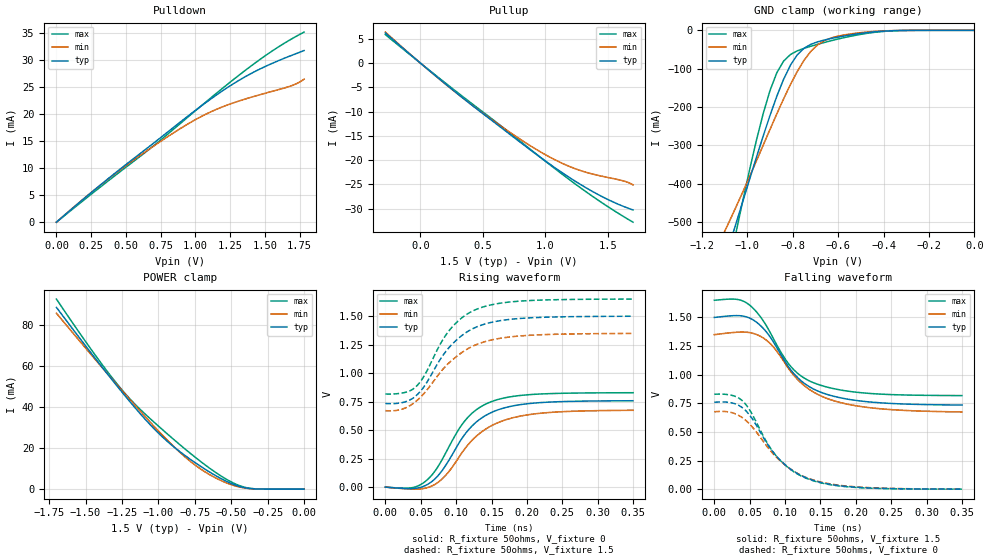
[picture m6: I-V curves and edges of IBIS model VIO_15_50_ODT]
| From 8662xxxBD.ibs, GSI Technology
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[Model]   VIO_15_50_ODT
Model_type   I/O
Polarity   Non-Inverting
Vinl  =   0.5500V
Vinh  =   0.9500V
Vmeas =   0.75v
Rref  =   50
|  variable   typ   min   max
C_comp   3.0pF   2.5pF   3.5pF
[Receiver Thresholds]
Vth = 0.75V
Vth_min = 0.68V
Vth_max = 0.825V
Threshold_sensitivity = 1.0
Reference_supply Ext_ref
Vinh_ac = +200mv
Vinh_dc = +100mv
Vinl_ac = -200mv
Vinl_dc = -100mv
Tslew_ac = 550ps
|  variable   typ   min   max
[External Reference]   0.75   0.68   0.825
|  variable   typ   min   max
[Temperature Range]   50   100   0
|  variable   typ   min   max
[Voltage Range]   1.5   1.35   1.65
[Add Submodel]
| Submodel Name   Mode
Strong_ODT_18V   Non-Driving
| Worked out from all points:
|   slope of the pulldown table from 0 to 0.225 V, typ, clamps not added: 45.5 ohm
|   slope of the pullup table from 0 to 0.225 V, typ, clamps not added: 46.7 ohm
|   GND clamp passes 1 mA (typ) near -0.36 V on its own axis
|   POWER clamp passes 1 mA (typ) near -0.42 V on its own axis
|   rising waveform, R_fixture 50ohms, V_fixture 0: 20-80 % time 55.1ps typ, 60.6ps min, 52.3ps max; typ from 0 V to 0.757 V
|   rising waveform, R_fixture 50ohms, V_fixture 1.5: 20-80 % time 56.4ps typ, 63.8ps min, 52.1ps max; typ from 0.733 V to 1.5 V
|   falling waveform, R_fixture 50ohms, V_fixture 1.5: 20-80 % time 59.4ps typ, 65.4ps min, 56ps max; typ from 1.5 V to 0.735 V
|   falling waveform, R_fixture 50ohms, V_fixture 0: 20-80 % time 58.8ps typ, 64.2ps min, 56.4ps max; typ from 0.759 V to 0 V
[Pullup]
| V(VDDQ-Vout)   typ   min   max
-280mV    6.194mA    6.382mA    5.865mA
40mV      -869.6uA   -882.7uA   -829.9uA
340mV     -7.204mA   -7.213mA   -6.928mA
620mV     -12.79mA   -12.56mA   -12.46mA
900mV     -18.3mA    -17.38mA   -18.2mA
1.08V     -21.65mA   -19.99mA   -21.84mA
1.24V     -24.38mA   -21.79mA   -24.95mA
1.34V     -25.93mA   -22.62mA   -26.8mA
1.48V     -27.87mA   -23.47mA   -29.27mA
1.62V     -29.5mA    -24.26mA   -31.56mA
1.7V      -30.27mA   -25.11mA   -32.79mA
[PullDown]
| voltage   typ   min   max
0V        -6.62nA    -14.14nA   -2.867nA
252mV     5.521mA    5.53mA     5.214mA
468mV     10.03mA    9.889mA    9.552mA
774mV     16.17mA    15.4mA     15.75mA
972mV     20.17mA    18.6mA     20.04mA
1.152V    23.59mA    20.93mA    23.91mA
1.368V    27.1mA     22.9mA     28.32mA
1.53V     29.18mA    24.1mA     31.34mA
1.674V    30.74mA    25.14mA    33.7mA
1.728V    31.28mA    25.68mA    34.49mA
1.782V    31.82mA    26.51mA    35.24mA
[POWER Clamp]
|V(VDDQ-Vout)   typ   min   max
-1.7V     88.47mA    85.63mA    92.51mA
-1.428V   63.15mA    62.67mA    64.71mA
-1.224V   45.01mA    45.89mA    46.19mA
-1.122V   36.5mA     37.74mA    38.64mA
-1.02V    28.71mA    29.85mA    31.98mA
-918mV    21.99mA    22.38mA    25.61mA
-816mV    16.3mA     15.63mA    19.48mA
-646mV    8.221mA    6.972mA    10.07mA
-544mV    4.192mA    3.378mA    5.259mA
-442mV    1.292mA    1.001mA    1.675mA
-340mV    147uA      124.8uA    177uA
0V        29.63nA    52.34nA    12.42nA
[GND Clamp]
|(Vout)   typ   min   max
-1.5V     -1.252A    -991.4mA   -1.695A
-1.11V    -618mA     -537.1mA   -698.9mA
-1.08V    -561.6mA   -499.5mA   -613mA
-1.05V    -504.3mA   -461mA     -527.9mA
-930mV    -275.4mA   -299.5mA   -216.7mA
-900mV    -221.7mA   -258.3mA   -156.7mA
-870mV    -171.8mA   -217.7mA   -110.4mA
-810mV    -90.75mA   -141.1mA   -63.05mA
-720mV    -36.4mA    -54.51mA   -41.47mA
-630mV    -21.2mA    -19.75mA   -26.98mA
-390mV    -1.825mA   -1.274mA   -2.426mA
0V        -6.62nA    -14.14nA   -2.873nA
[Ramp]
| voltage   typ   min   max
dV/dt_r   0.54/186p   0.48/213p   0.60/209p
dV/dt_f   0.86/129p   0.66/166p   1.07/101p
R_load  =   50ohms
[Rising Waveform]
R_fixture =   50ohms
V_fixture =   0
| Time   V(typ)   V(min)   V(max)
0s        156.2nV    330.9nV    69.99nV
38.5ps    -12.6mV    -17.51mV   -3.974mV
63ps      37.07mV    2.813mV    87.25mV
84ps      178.8mV    95.17mV    284.9mV
112ps     460.4mV    333.9mV    578.9mV
129.5ps   575.8mV    451.7mV    682.8mV
150.5ps   656.1mV    540.2mV    750.9mV
178.5ps   710mV      605.5mV    793.7mV
217ps     740.1mV    646.3mV    815.9mV
350ps     757.4mV    673.7mV    827.7mV
[Rising Waveform]
R_fixture =   50ohms
V_fixture =   1.5
V_fixture_min =  1.35
V_fixture_max =  1.65
| Time   V(typ)   V(min)   V(max)
0s        733.1mV    670.5mV    816.7mV
21ps      737.8mV    679mV      822.5mV
42ps      793.7mV    745.8mV    873.6mV
52.5ps    862.7mV    806.5mV    951.4mV
77ps      1.115V     1.001V     1.247V
91ps      1.231V     1.096V     1.379V
112ps     1.347V     1.196V     1.503V
133ps     1.414V     1.26V      1.569V
199.5ps   1.482V     1.329V     1.634V
350ps     1.498V     1.347V     1.649V
[Falling Waveform]
R_fixture =   50ohms
V_fixture =   1.5
V_fixture_min = 1.35
V_fixture_max = 1.65
| Time   V(typ)   V(min)   V(max)
0s        1.5V       1.35V      1.65V
35ps      1.516V     1.372V     1.654V
59.5ps    1.459V     1.351V     1.549V
80.5ps    1.315V     1.262V     1.351V
105ps     1.067V     1.052V     1.094V
122.5ps   947.5mV    928.9mV    989.3mV
140ps     875.3mV    848.7mV    930.3mV
168ps     812.7mV    774mV      879mV
210ps     767.8mV    719.4mV    841.2mV
350ps     735mV      674.7mV    817.5mV
[Falling Waveform]
R_fixture =   50ohms
V_fixture =   0
| Time   V(typ)   V(min)   V(max)
0s        759.1mV    676.3mV    828.8mV
21ps      757.9mV    673.9mV    824.3mV
38.5ps    717.2mV    629.2mV    778.6mV
52.5ps    625.1mV    551.5mV    665.6mV
73.5ps    408.9mV    381.1mV    416.6mV
87.5ps    290.5mV    280.5mV    289.9mV
108.5ps   172.1mV    172.4mV    168.7mV
133ps     91.44mV    94.65mV    88.25mV
199.5ps   17.81mV    20.79mV    15.6mV
350ps     497.4uV    868.6uV    301.1uV
